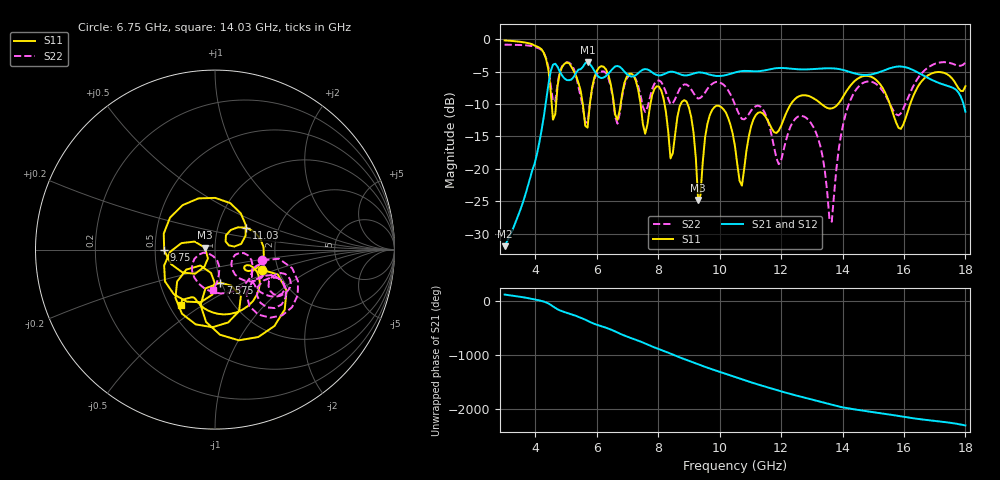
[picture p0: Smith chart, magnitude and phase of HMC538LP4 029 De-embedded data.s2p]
! Chelmsford, MA 01824
! http://www.hittite.com
! Tel: 978-250-3343
! Fax: 978-250-3373
! Device  :  HMC538LP4
! Description:  600 Analog Phase Shifter
! Frequency  :  6.0 GHz - 15.0 GHz
! Package  :  LP4  - 4x4 mm Quad Flatpack No-Lead (QFN) Plastic Package: 24 pin
! Ports  :  2 RF, 1 DC
!  Pin  3  = Rfin  = Port 1
!  Pin  16  = Rfout = Port 2
!  pin  21  = vCTL
! Voltages:  VCTL  = 0 to 5.0 Volts
! Currents :  Vb(V)  Vd(V)  Ib(mA)  Id(mA)
!  0.00  2.90  0.000000	0.465805
! Data:  The device was measured on evaluation board 111296-1.
!  Data was collected using a calibrated network analyzer.
!  The evaluation circuit board was modeled and simulated.This was use
!  to removed the evaluation board circuit from the measured data.
!  The reference plane is the center of the package pin.
! Misc:  Lot #
!Date Measured:  03 - 11 -2009
! Date:  03 - 17 -2009
! Note:
!  Hittite Microwave supplies this data as a sample of measured data at the
!  package pin for this package product.  Your particular data for this product
!  may vary.
!  Data was taken at 25 degrees C.
!  Hittite Microwave reserves the right to change this data at anytime.
# MHz S MA R 50
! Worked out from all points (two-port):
!   201 points, 3 GHz to 18 GHz, reference 50 ohm
!   highest |S21| = -3.55 dB at 5.7 GHz (marker M1); lowest = -31.9 dB at 3 GHz (marker M2)
!   |S21| within 3 dB of the highest: 4.442 GHz to 17.03 GHz (12.59 GHz wide, 117 % of centre)
!   lowest |S11| = -24.8 dB at 9.3 GHz (marker M3), VSWR 1.12, Z = 44.6 + j0.947 ohm
!   |S11| at or under -10 dB: 8.206 GHz to 8.736 GHz (530.1 MHz wide, 6.26 % of centre); 8.955 GHz to 12.32 GHz (3.366 GHz wide, 31.6 % of centre); 15.54 GHz to 16.2 GHz (664.1 MHz wide, 4.18 % of centre)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
!   |S22| runs from -28.1 to -0.9 dB; largest |S21 - S12| = 0.0025
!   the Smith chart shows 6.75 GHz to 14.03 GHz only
!   S11 on the Smith chart (normalised r, x): 6.75 GHz: 1.65, -0.40; 7.575 GHz: 0.99, -0.38; 9.75 GHz: 0.56, -0.01; 11.03 GHz: 1.37, +0.35; 14.03 GHz: 0.58, -0.41
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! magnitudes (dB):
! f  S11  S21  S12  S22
! 3 GHz  -0.2  -31.9  -31.9  -0.9
! 4.275 GHz  -2.1  -12.0  -12.0  -2.1
! 4.575 GHz  -12.4  -3.9  -3.9  -9.6
! 5.025 GHz  -3.6  -6.3  -6.3  -3.6
! 5.55 GHz  -10.2  -4.3  -4.3  -10.7
! 5.7 GHz  -13.6  -3.5  -3.6  -12.9
! 6.15 GHz  -4.2  -6.0  -6.0  -5.0
! 6.75 GHz  -10.9  -4.3  -4.3  -11.4
! 7.575 GHz  -14.6  -4.6  -4.6  -11.2
! 8.025 GHz  -7.3  -5.6  -5.6  -6.4
! 8.4 GHz  -18.4  -5.0  -5.0  -10.0
! 9 GHz  -10.5  -5.5  -5.5  -7.3
! 9.3 GHz  -24.8  -5.1  -5.1  -9.2
! 9.75 GHz  -11.0  -5.6  -5.6  -6.9
! 10.5 GHz  -16.5  -5.1  -5.2  -10.1
! 10.72 GHz  -22.6  -4.9  -4.9  -12.3
! 11.03 GHz  -13.4  -4.9  -4.9  -11.0
! 13.05 GHz  -9.1  -4.6  -4.6  -13.5
! 13.65 GHz  -10.7  -4.5  -4.5  -28.1
! 14.03 GHz  -8.8  -4.8  -4.8  -13.1
! 15.53 GHz  -9.8  -4.5  -4.5  -9.8
! 18 GHz  -7.3  -11.2  -11.2  -3.6
